| IBIS file stm32u575_585_lqfp144.ibs
[IBIS ver] 4.2
[File name] stm32u575_585_lqfp144.ibs
[File Rev] 1.0
[Date]   06-08-2021
[Source] Data Created at STMicroelectronics
[Notes]  File originated from ELDO simulations.
[Disclaimer]  This information is for modeling purpose only and is
   not guaranted. The information is subject to change without
   notice.
[Copyright] Copyright 2021 STMicroelectronics Inc.
|   Component stm32u575_585_lqfp144
[Component] stm32u575_585_lqfp144
[Manufacturer] STMicroelectronics
[Package]
| variable   typ   min   max
R_pkg   0   NA   NA
L_pkg   0   NA   NA
C_pkg   0   NA   NA
[Pin]   signal_name   model_name   R_pin   L_pin   C_pin   | Comment
1 PE2 io8_100m_hslv_ft 187.6E-3 9.4E-9 267.9E-15
2 PE3 io8_100m_hslv_tamp_ft 182.4E-3 9.1E-9 243.8E-15
3 PE4 io8_100m_hslv_tamp_ft 177.6E-3 8.7E-9 221.3E-15
4 PE5 io8_100m_hslv_tamp_ft 173.1E-3 8.4E-9 200.2E-15
5 PE6 io8_100m_hslv_tamp_ft 168.9E-3 8.1E-9 180.5E-15
6 VBAT POWER 165.0E-3 7.8E-9 162.3E-15
7 PC13 io8_100m_ft_v33 161.5E-3 7.6E-9 145.6E-15
8 PC14-OSC32_IN io8_100m_ft 158.2E-3 7.4E-9 130.3E-15
9 PC15-OSC32_OUT io8_100m_ft 155.2E-3 7.2E-9 116.4E-15
10 PF0 io8_100m_hslv_ft 152.6E-3 7.0E-9 104.1E-15
11 PF1 io8_100m_hslv_ft 150.3E-3 6.8E-9 93.2E-15
12 PF2 io8_100m_hslv_ft 148.2E-3 6.7E-9 83.7E-15
13 PF3 io8_100m_hslv_ft 146.5E-3 6.5E-9 75.7E-15
14 PF4 io8_166m_hslv_ft 145.1E-3 6.4E-9 69.1E-15
15 PF5 io8_166m_hslv_ft 144.1E-3 6.4E-9 64.0E-15
16 VSS GND 143.3E-3 6.3E-9 60.4E-15
17 VDD POWER 142.8E-3 6.3E-9 58.2E-15
18 PF6 io8_100m_hslv_ft 142.7E-3 6.3E-9 57.5E-15
19 PF7 io8_100m_hslv_ft 142.7E-3 6.3E-9 57.5E-15
20 PF8 io8_100m_hslv_ft 142.8E-3 6.3E-9 58.2E-15
21 PF9 io8_100m_hslv_ft 143.3E-3 6.3E-9 60.4E-15
22 PF10 io8_166m_hslv_ft 144.1E-3 6.4E-9 64.0E-15
23 PH0-OSC_IN io8_100m_ft 145.1E-3 6.4E-9 69.1E-15
24 PH1-OSC_OUT io8_100m_ft 146.5E-3 6.5E-9 75.7E-15
25 NRST nc 148.2E-3 6.7E-9 83.7E-15
26 PC0 io8_100m_hslv_ft 150.3E-3 6.8E-9 93.2E-15
27 PC1 io8_166m_hslv_i2c_ft 152.6E-3 7.0E-9 104.1E-15
28 PC2 io8_100m_hslv_ft 155.2E-3 7.2E-9 116.4E-15
29 PC3 io8_100m_hslv_ft 158.2E-3 7.4E-9 130.3E-15
30 VSSA GND 161.5E-3 7.6E-9 145.6E-15
31 VREF- GND 165.0E-3 7.8E-9 162.3E-15
32 VREF+ POWER 168.9E-3 8.1E-9 180.5E-15
33 VDDA POWER 173.1E-3 8.4E-9 200.2E-15
34 PA0 io8_100m_hslv_tamp_ft 177.6E-3 8.7E-9 221.3E-15
35 PA1 io8_100m_hslv_tamp_ft 182.4E-3 9.1E-9 243.8E-15
36 PA2 io8_100m_hslv_ft 187.6E-3 9.4E-9 267.9E-15
37 PA3 io8_166m_hslv_ft 187.6E-3 9.4E-9 267.9E-15
38 VSS GND 182.4E-3 9.1E-9 243.8E-15
39 VDD POWER 177.6E-3 8.7E-9 221.3E-15
40 PA4 io8_100m_hslv_ft 173.1E-3 8.4E-9 200.2E-15
41 PA5 io8_100m_ft 168.9E-3 8.1E-9 180.5E-15
42 PA6 io8_100m_hslv_ft 165.0E-3 7.8E-9 162.3E-15
43 PA7 io8_100m_hslv_ft 161.5E-3 7.6E-9 145.6E-15
44 PC4 io8_100m_hslv_ft 158.2E-3 7.4E-9 130.3E-15
45 PC5 io8_100m_tamp_ft 155.2E-3 7.2E-9 116.4E-15
46 PB0 io8_100m_hslv_ft 152.6E-3 7.0E-9 104.1E-15
47 PB1 io8_100m_hslv_ft 150.3E-3 6.8E-9 93.2E-15
48 PB2 io8_100m_hslv_tamp_ft 148.2E-3 6.7E-9 83.7E-15
49 PF11 io8_166m_hslv_ft 146.5E-3 6.5E-9 75.7E-15
50 PF12 io8_100m_hslv_ft 145.1E-3 6.4E-9 69.1E-15
51 VSS GND 144.1E-3 6.4E-9 64.0E-15
52 VDD POWER 143.3E-3 6.3E-9 60.4E-15
53 PF13 io8_100m_hslv_ft 142.8E-3 6.3E-9 58.2E-15
54 PF14 io8_100m_hslv_ft 142.7E-3 6.3E-9 57.5E-15
55 PF15 io8_100m_hslv_ft 142.7E-3 6.3E-9 57.5E-15
56 PG0 io8_100m_hslv_ft 142.8E-3 6.3E-9 58.2E-15
57 PG1 io8_100m_hslv_ft 143.3E-3 6.3E-9 60.4E-15
58 PE7 io8_100m_hslv_ft 144.1E-3 6.4E-9 64.0E-15
59 PE8 io8_100m_hslv_ft 145.1E-3 6.4E-9 69.1E-15
60 PE9 io8_166m_hslv_ft 146.5E-3 6.5E-9 75.7E-15
61 VSS GND 148.2E-3 6.7E-9 83.7E-15
62 VDD POWER 150.3E-3 6.8E-9 93.2E-15
63 PE10 io8_166m_hslv_ft 152.6E-3 7.0E-9 104.1E-15
64 PE11 io8_100m_hslv_ft 155.2E-3 7.2E-9 116.4E-15
65 PE12 io8_100m_hslv_ft 158.2E-3 7.4E-9 130.3E-15
66 PE13 io8_100m_hslv_ft 161.5E-3 7.6E-9 145.6E-15
67 PE14 io8_100m_hslv_ft 165.0E-3 7.8E-9 162.3E-15
68 PE15 io8_100m_hslv_ft 168.9E-3 8.1E-9 180.5E-15
69 PB10 io8_166m_hslv_i2c_ft 173.1E-3 8.4E-9 200.2E-15
70 VCAP POWER 177.6E-3 8.7E-9 221.3E-15
71 VSS GND 182.4E-3 9.1E-9 243.8E-15
72 VDD POWER 187.6E-3 9.4E-9 267.9E-15
73 PB12 io8_166m_hslv_ft 187.6E-3 9.4E-9 267.9E-15
74 PB13 io8_100m_i2c_ft 182.4E-3 9.1E-9 243.8E-15
75 PB14 io8_100m_i2c_ft 177.6E-3 8.7E-9 221.3E-15
76 PB15 nc 173.1E-3 8.4E-9 200.2E-15
77 PD8 io8_100m_hslv_ft 168.9E-3 8.1E-9 180.5E-15
78 PD9 io8_100m_hslv_ft 165.0E-3 7.8E-9 162.3E-15
79 PD10 io8_100m_hslv_ft 161.5E-3 7.6E-9 145.6E-15
80 PD11 io8_100m_hslv_ft 158.2E-3 7.4E-9 130.3E-15
81 PD12 io8_100m_hslv_ft 155.2E-3 7.2E-9 116.4E-15
82 PD13 io8_100m_hslv_ft 152.6E-3 7.0E-9 104.1E-15
83 VSS GND 150.3E-3 6.8E-9 93.2E-15
84 VDD POWER 148.2E-3 6.7E-9 83.7E-15
85 PD14 io8_100m_hslv_ft 146.5E-3 6.5E-9 75.7E-15
86 PD15 io8_100m_hslv_ft 145.1E-3 6.4E-9 69.1E-15
87 PG2 io8_100m_hslv_ft 144.1E-3 6.4E-9 64.0E-15
88 PG3 io8_100m_hslv_ft 143.3E-3 6.3E-9 60.4E-15
89 PG4 io8_100m_hslv_ft 142.8E-3 6.3E-9 58.2E-15
90 PG5 io8_100m_hslv_ft 142.7E-3 6.3E-9 57.5E-15
91 PG6 io8_100m_hslv_ft 142.7E-3 6.3E-9 57.5E-15
92 PG7 io8_100m_hslv_ft 142.8E-3 6.3E-9 58.2E-15
93 PG8 io8_100m_i2c_ft 143.3E-3 6.3E-9 60.4E-15
94 VSS GND 144.1E-3 6.4E-9 64.0E-15
95 VDDIO2 POWER 145.1E-3 6.4E-9 69.1E-15
96 PC6 io8_100m_ft 146.5E-3 6.5E-9 75.7E-15
97 PC7 io8_100m_ft 148.2E-3 6.7E-9 83.7E-15
98 PC8 io8_100m_ft 150.3E-3 6.8E-9 93.2E-15
99 PC9 io8_100m_ft 152.6E-3 7.0E-9 104.1E-15
100 PA8 io8_166m_hslv_ft 155.2E-3 7.2E-9 116.4E-15
101 PA9 io8_100m_usb_vbus_ft 158.2E-3 7.4E-9 130.3E-15
102 PA10 io8_100m_usb_id 161.5E-3 7.6E-9 145.6E-15
103 PA11 io8_usb_ft 165.0E-3 7.8E-9 162.3E-15
104 PA12 io8_usb_ft 168.9E-3 8.1E-9 180.5E-15
105 PA13 io8_100m_ft 173.1E-3 8.4E-9 200.2E-15
106 VDDUSB POWER 177.6E-3 8.7E-9 221.3E-15
107 VSS GND 182.4E-3 9.1E-9 243.8E-15
108 VDD POWER 187.6E-3 9.4E-9 267.9E-15
109 PA14 io8_100m_ft 187.6E-3 9.4E-9 267.9E-15
110 PA15 nc 182.4E-3 9.1E-9 243.8E-15
111 PC10 io8_100m_ft 177.6E-3 8.7E-9 221.3E-15
112 PC11 io8_100m_hslv_ft 173.1E-3 8.4E-9 200.2E-15
113 PC12 io8_166m_hslv_ft 168.9E-3 8.1E-9 180.5E-15
114 PD0 io8_100m_hslv_ft 165.0E-3 7.8E-9 162.3E-15
115 PD1 io8_100m_hslv_ft 161.5E-3 7.6E-9 145.6E-15
116 PD2 io8_100m_ft 158.2E-3 7.4E-9 130.3E-15
117 PD3 io8_166m_hslv_ft 155.2E-3 7.2E-9 116.4E-15
118 PD4 io8_100m_hslv_ft 152.6E-3 7.0E-9 104.1E-15
119 PD5 io8_100m_hslv_ft 150.3E-3 6.8E-9 93.2E-15
120 VSS GND 148.2E-3 6.7E-9 83.7E-15
121 VDD POWER 146.5E-3 6.5E-9 75.7E-15
122 PD6 io8_166m_hslv_ft 145.1E-3 6.4E-9 69.1E-15
123 PD7 io8_100m_hslv_ft 144.1E-3 6.4E-9 64.0E-15
124 PG9 io8_100m_hslv_ft 143.3E-3 6.3E-9 60.4E-15
125 PG10 io8_100m_hslv_ft 142.8E-3 6.3E-9 58.2E-15
126 PG11 io8_100m_hslv_ft 142.7E-3 6.3E-9 57.5E-15
127 PG12 io8_100m_hslv_ft 142.7E-3 6.3E-9 57.5E-15
128 PG13 io8_100m_hslv_ft 142.8E-3 6.3E-9 58.2E-15
129 PG14 io8_100m_hslv_ft 143.3E-3 6.3E-9 60.4E-15
130 VSS GND 144.1E-3 6.4E-9 64.0E-15
131 VDDIO2 POWER 145.1E-3 6.4E-9 69.1E-15
132 PG15 io8_100m_hslv_ft 146.5E-3 6.5E-9 75.7E-15
133 PB3 io8_100m_i2c_ft 148.2E-3 6.7E-9 83.7E-15
134 PB4 io8_100m_i2c_ft 150.3E-3 6.8E-9 93.2E-15
135 PB5 io8_166m_hslv_ft 152.6E-3 7.0E-9 104.1E-15
136 PB6 io8_100m_i2c_ft 155.2E-3 7.2E-9 116.4E-15
137 PB7 io8_166m_hslv_i2c_ft 158.2E-3 7.4E-9 130.3E-15
138 PH3-BOOT0 io8_100m_ft 161.5E-3 7.6E-9 145.6E-15
139 PB8 io8_100m_i2c_ft 165.0E-3 7.8E-9 162.3E-15
140 PB9 io8_100m_i2c_ft 168.9E-3 8.1E-9 180.5E-15
141 PE0 io8_100m_hslv_ft 173.1E-3 8.4E-9 200.2E-15
142 PE1 io8_100m_hslv_ft 177.6E-3 8.7E-9 221.3E-15
143 VSS GND 182.4E-3 9.1E-9 243.8E-15
144 VDD POWER 187.6E-3 9.4E-9 267.9E-15
[Model Selector] io8_100m_ft
io8_100m_ft_hs_1v2  "IO8_FT 100MHz high speed @ 1.2V"
io8_100m_ft_hs_pu_1v2  "IO8_FT 100MHz high speed @ 1.2V pullup"
io8_100m_ft_hs_pd_1v2  "IO8_FT 100MHz high speed @ 1.2V pulldown"
io8_100m_ft_fs_1v2  "IO8_FT 100MHz fast speed @ 1.2V"
io8_100m_ft_fs_pu_1v2  "IO8_FT 100MHz fast speed @ 1.2V pullup"
io8_100m_ft_fs_pd_1v2  "IO8_FT 100MHz fast speed @ 1.2V pulldown"
io8_100m_ft_ms_1v2  "IO8_FT 100MHz med speed @ 1.2V"
io8_100m_ft_ms_pu_1v2  "IO8_FT 100MHz med speed @ 1.2V pullup"
io8_100m_ft_ms_pd_1v2  "IO8_FT 100MHz med speed @ 1.2V pulldown"
io8_100m_ft_ls_1v2  "IO8_FT 100MHz low speed @ 1.2V"
io8_100m_ft_ls_pu_1v2  "IO8_FT 100MHz low speed @ 1.2V pullup"
io8_100m_ft_ls_pd_1v2  "IO8_FT 100MHz low speed @ 1.2V pulldown"
io8_100m_ft_hs_1v8  "IO8_FT 100MHz high speed @ 1.8V"
io8_100m_ft_hs_pu_1v8  "IO8_FT 100MHz high speed @ 1.8V pullup"
io8_100m_ft_hs_pd_1v8  "IO8_FT 100MHz high speed @ 1.8V pulldown"
io8_100m_ft_fs_1v8  "IO8_FT 100MHz fast speed @ 1.8V"
io8_100m_ft_fs_pu_1v8  "IO8_FT 100MHz fast speed @ 1.8V pullup"
io8_100m_ft_fs_pd_1v8  "IO8_FT 100MHz fast speed @ 1.8V pulldown"
io8_100m_ft_ms_1v8  "IO8_FT 100MHz med speed @ 1.8V"
io8_100m_ft_ms_pu_1v8  "IO8_FT 100MHz med speed @ 1.8V pullup"
io8_100m_ft_ms_pd_1v8  "IO8_FT 100MHz med speed @ 1.8V pulldown"
io8_100m_ft_ls_1v8  "IO8_FT 100MHz low speed @ 1.8V"
io8_100m_ft_ls_pu_1v8  "IO8_FT 100MHz low speed @ 1.8V pullup"
io8_100m_ft_ls_pd_1v8  "IO8_FT 100MHz low speed @ 1.8V pulldown"
io8_100m_ft_hs_3v3  "IO8_FT 100MHz high speed @ 3.3V"
io8_100m_ft_hs_pu_3v3  "IO8_FT 100MHz high speed @ 3.3V pullup"
io8_100m_ft_hs_pd_3v3  "IO8_FT 100MHz high speed @ 3.3V pulldown"
io8_100m_ft_fs_3v3  "IO8_FT 100MHz fast speed @ 3.3V"
io8_100m_ft_fs_pu_3v3  "IO8_FT 100MHz fast speed @ 3.3V pullup"
io8_100m_ft_fs_pd_3v3  "IO8_FT 100MHz fast speed @ 3.3V pulldown"
io8_100m_ft_ms_3v3  "IO8_FT 100MHz med speed @ 3.3V"
io8_100m_ft_ms_pu_3v3  "IO8_FT 100MHz med speed @ 3.3V pullup"
io8_100m_ft_ms_pd_3v3  "IO8_FT 100MHz med speed @ 3.3V pulldown"
io8_100m_ft_ls_3v3  "IO8_FT 100MHz low speed @ 3.3V"
io8_100m_ft_ls_pu_3v3  "IO8_FT 100MHz low speed @ 3.3V pullup"
io8_100m_ft_ls_pd_3v3  "IO8_FT 100MHz low speed @ 3.3V pulldown"
[Model Selector] io8_100m_hslv_ft
io8_100m_ft_hs_1v2  "IO8_FT 100MHz high speed @ 1.2V"
io8_100m_ft_hs_pu_1v2  "IO8_FT 100MHz high speed @ 1.2V pullup"
io8_100m_ft_hs_pd_1v2  "IO8_FT 100MHz high speed @ 1.2V pulldown"
io8_100m_ft_fs_1v2  "IO8_FT 100MHz fast speed @ 1.2V"
io8_100m_ft_fs_pu_1v2  "IO8_FT 100MHz fast speed @ 1.2V pullup"
io8_100m_ft_fs_pd_1v2  "IO8_FT 100MHz fast speed @ 1.2V pulldown"
io8_100m_ft_ms_1v2  "IO8_FT 100MHz med speed @ 1.2V"
io8_100m_ft_ms_pu_1v2  "IO8_FT 100MHz med speed @ 1.2V pullup"
io8_100m_ft_ms_pd_1v2  "IO8_FT 100MHz med speed @ 1.2V pulldown"
io8_100m_ft_ls_1v2  "IO8_FT 100MHz low speed @ 1.2V"
io8_100m_ft_ls_pu_1v2  "IO8_FT 100MHz low speed @ 1.2V pullup"
io8_100m_ft_ls_pd_1v2  "IO8_FT 100MHz low speed @ 1.2V pulldown"
io8_100m_ft_hs_1v8  "IO8_FT 100MHz high speed @ 1.8V"
io8_100m_ft_hs_pu_1v8  "IO8_FT 100MHz high speed @ 1.8V pullup"
io8_100m_ft_hs_pd_1v8  "IO8_FT 100MHz high speed @ 1.8V pulldown"
io8_100m_ft_fs_1v8  "IO8_FT 100MHz fast speed @ 1.8V"
io8_100m_ft_fs_pu_1v8  "IO8_FT 100MHz fast speed @ 1.8V pullup"
io8_100m_ft_fs_pd_1v8  "IO8_FT 100MHz fast speed @ 1.8V pulldown"
io8_100m_ft_ms_1v8  "IO8_FT 100MHz med speed @ 1.8V"
io8_100m_ft_ms_pu_1v8  "IO8_FT 100MHz med speed @ 1.8V pullup"
io8_100m_ft_ms_pd_1v8  "IO8_FT 100MHz med speed @ 1.8V pulldown"
io8_100m_ft_ls_1v8  "IO8_FT 100MHz low speed @ 1.8V"
io8_100m_ft_ls_pu_1v8  "IO8_FT 100MHz low speed @ 1.8V pullup"
io8_100m_ft_ls_pd_1v8  "IO8_FT 100MHz low speed @ 1.8V pulldown"
io8_100m_ft_hs_3v3  "IO8_FT 100MHz high speed @ 3.3V"
io8_100m_ft_hs_pu_3v3  "IO8_FT 100MHz high speed @ 3.3V pullup"
io8_100m_ft_hs_pd_3v3  "IO8_FT 100MHz high speed @ 3.3V pulldown"
io8_100m_ft_fs_3v3  "IO8_FT 100MHz fast speed @ 3.3V"
io8_100m_ft_fs_pu_3v3  "IO8_FT 100MHz fast speed @ 3.3V pullup"
io8_100m_ft_fs_pd_3v3  "IO8_FT 100MHz fast speed @ 3.3V pulldown"
io8_100m_ft_ms_3v3  "IO8_FT 100MHz med speed @ 3.3V"
io8_100m_ft_ms_pu_3v3  "IO8_FT 100MHz med speed @ 3.3V pullup"
io8_100m_ft_ms_pd_3v3  "IO8_FT 100MHz med speed @ 3.3V pulldown"
io8_100m_ft_ls_3v3  "IO8_FT 100MHz low speed @ 3.3V"
io8_100m_ft_ls_pu_3v3  "IO8_FT 100MHz low speed @ 3.3V pullup"
io8_100m_ft_ls_pd_3v3  "IO8_FT 100MHz low speed @ 3.3V pulldown"
io8_100m_hslv_ft_hs_1v2  "IO8_FT 100MHz HSLV high speed @ 1.2V"
io8_100m_hslv_ft_hs_pu_1v2  "IO8_FT 100MHz HSLV high speed @ 1.2V pullup"
io8_100m_hslv_ft_hs_pd_1v2  "IO8_FT 100MHz HSLV high speed @ 1.2V pulldown"
io8_100m_hslv_ft_fs_1v2  "IO8_FT 100MHz HSLV fast speed @ 1.2V"
io8_100m_hslv_ft_fs_pu_1v2  "IO8_FT 100MHz HSLV fast speed @ 1.2V pullup"
io8_100m_hslv_ft_fs_pd_1v2  "IO8_FT 100MHz HSLV fast speed @ 1.2V pulldown"
io8_100m_hslv_ft_ms_1v2  "IO8_FT 100MHz HSLV med speed @ 1.2V"
io8_100m_hslv_ft_ms_pu_1v2  "IO8_FT 100MHz HSLV med speed @ 1.2V pullup"
io8_100m_hslv_ft_ms_pd_1v2  "IO8_FT 100MHz HSLV med speed @ 1.2V pulldown"
io8_100m_hslv_ft_ls_1v2  "IO8_FT 100MHz HSLV low speed @ 1.2V"
io8_100m_hslv_ft_ls_pu_1v2  "IO8_FT 100MHz HSLV low speed @ 1.2V pullup"
io8_100m_hslv_ft_ls_pd_1v2  "IO8_FT 100MHz HSLV low speed @ 1.2V pulldown"
io8_100m_hslv_ft_hs_1v8  "IO8_FT 100MHz HSLV high speed @ 1.8V"
io8_100m_hslv_ft_hs_pu_1v8  "IO8_FT 100MHz HSLV high speed @ 1.8V pullup"
io8_100m_hslv_ft_hs_pd_1v8  "IO8_FT 100MHz HSLV high speed @ 1.8V pulldown"
io8_100m_hslv_ft_fs_1v8  "IO8_FT 100MHz HSLV fast speed @ 1.8V"
io8_100m_hslv_ft_fs_pu_1v8  "IO8_FT 100MHz HSLV fast speed @ 1.8V pullup"
io8_100m_hslv_ft_fs_pd_1v8  "IO8_FT 100MHz HSLV fast speed @ 1.8V pulldown"
io8_100m_hslv_ft_ms_1v8  "IO8_FT 100MHz HSLV med speed @ 1.8V"
io8_100m_hslv_ft_ms_pu_1v8  "IO8_FT 100MHz HSLV med speed @ 1.8V pullup"
io8_100m_hslv_ft_ms_pd_1v8  "IO8_FT 100MHz HSLV med speed @ 1.8V pulldown"
io8_100m_hslv_ft_ls_1v8  "IO8_FT 100MHz HSLV low speed @ 1.8V"
io8_100m_hslv_ft_ls_pu_1v8  "IO8_FT 100MHz HSLV low speed @ 1.8V pullup"
io8_100m_hslv_ft_ls_pd_1v8  "IO8_FT 100MHz HSLV low speed @ 1.8V pulldown"
io8_100m_hslv_ft_hs_2v5  "IO8_FT 100MHz HSLV high speed @ 2.5V"
io8_100m_hslv_ft_hs_pu_2v5  "IO8_FT 100MHz HSLV high speed @ 2.5V pullup"
io8_100m_hslv_ft_hs_pd_2v5  "IO8_FT 100MHz HSLV high speed @ 2.5V pulldown"
io8_100m_hslv_ft_fs_2v5  "IO8_FT 100MHz HSLV fast speed @ 2.5V"
io8_100m_hslv_ft_fs_pu_2v5  "IO8_FT 100MHz HSLV fast speed @ 2.5V pullup"
io8_100m_hslv_ft_fs_pd_2v5  "IO8_FT 100MHz HSLV fast speed @ 2.5V pulldown"
io8_100m_hslv_ft_ms_2v5  "IO8_FT 100MHz HSLV med speed @ 2.5V"
io8_100m_hslv_ft_ms_pu_2v5  "IO8_FT 100MHz HSLV med speed @ 2.5V pullup"
io8_100m_hslv_ft_ms_pd_2v5  "IO8_FT 100MHz HSLV med speed @ 2.5V pulldown"
io8_100m_hslv_ft_ls_2v5  "IO8_FT 100MHz HSLV low speed @ 2.5V"
io8_100m_hslv_ft_ls_pu_2v5  "IO8_FT 100MHz HSLV low speed @ 2.5V pullup"
io8_100m_hslv_ft_ls_pd_2v5  "IO8_FT 100MHz HSLV low speed @ 2.5V pulldown"
[Model Selector] io8_166m_hslv_ft
io8_166m_ft_hs_1v2  "IO8_FT 166MHz high speed @ 1.2V"
io8_166m_ft_hs_pu_1v2  "IO8_FT 166MHz high speed @ 1.2V pullup"
io8_166m_ft_hs_pd_1v2  "IO8_FT 166MHz high speed @ 1.2V pulldown"
io8_166m_ft_fs_1v2  "IO8_FT 166MHz fast speed @ 1.2V"
io8_166m_ft_fs_pu_1v2  "IO8_FT 166MHz fast speed @ 1.2V pullup"
io8_166m_ft_fs_pd_1v2  "IO8_FT 166MHz fast speed @ 1.2V pulldown"
io8_166m_ft_ms_1v2  "IO8_FT 166MHz med speed @ 1.2V"
io8_166m_ft_ms_pu_1v2  "IO8_FT 166MHz med speed @ 1.2V pullup"
io8_166m_ft_ms_pd_1v2  "IO8_FT 166MHz med speed @ 1.2V pulldown"
io8_166m_ft_ls_1v2  "IO8_FT 166MHz low speed @ 1.2V"
io8_166m_ft_ls_pu_1v2  "IO8_FT 166MHz low speed @ 1.2V pullup"
io8_166m_ft_ls_pd_1v2  "IO8_FT 166MHz low speed @ 1.2V pulldown"
io8_166m_ft_hs_1v8  "IO8_FT 166MHz high speed @ 1.8V"
io8_166m_ft_hs_pu_1v8  "IO8_FT 166MHz high speed @ 1.8V pullup"
io8_166m_ft_hs_pd_1v8  "IO8_FT 166MHz high speed @ 1.8V pulldown"
io8_166m_ft_fs_1v8  "IO8_FT 166MHz fast speed @ 1.8V"
io8_166m_ft_fs_pu_1v8  "IO8_FT 166MHz fast speed @ 1.8V pullup"
io8_166m_ft_fs_pd_1v8  "IO8_FT 166MHz fast speed @ 1.8V pulldown"
io8_166m_ft_ms_1v8  "IO8_FT 166MHz med speed @ 1.8V"
io8_166m_ft_ms_pu_1v8  "IO8_FT 166MHz med speed @ 1.8V pullup"
io8_166m_ft_ms_pd_1v8  "IO8_FT 166MHz med speed @ 1.8V pulldown"
io8_166m_ft_ls_1v8  "IO8_FT 166MHz low speed @ 1.8V"
io8_166m_ft_ls_pu_1v8  "IO8_FT 166MHz low speed @ 1.8V pullup"
io8_166m_ft_ls_pd_1v8  "IO8_FT 166MHz low speed @ 1.8V pulldown"
io8_166m_ft_hs_3v3  "IO8_FT 166MHz high speed @ 3.3V"
io8_166m_ft_hs_pu_3v3  "IO8_FT 166MHz high speed @ 3.3V pullup"
io8_166m_ft_hs_pd_3v3  "IO8_FT 166MHz high speed @ 3.3V pulldown"
io8_166m_ft_fs_3v3  "IO8_FT 166MHz fast speed @ 3.3V"
io8_166m_ft_fs_pu_3v3  "IO8_FT 166MHz fast speed @ 3.3V pullup"
io8_166m_ft_fs_pd_3v3  "IO8_FT 166MHz fast speed @ 3.3V pulldown"
io8_166m_ft_ms_3v3  "IO8_FT 166MHz med speed @ 3.3V"
io8_166m_ft_ms_pu_3v3  "IO8_FT 166MHz med speed @ 3.3V pullup"
io8_166m_ft_ms_pd_3v3  "IO8_FT 166MHz med speed @ 3.3V pulldown"
io8_166m_ft_ls_3v3  "IO8_FT 166MHz low speed @ 3.3V"
io8_166m_ft_ls_pu_3v3  "IO8_FT 166MHz low speed @ 3.3V pullup"
io8_166m_ft_ls_pd_3v3  "IO8_FT 166MHz low speed @ 3.3V pulldown"
io8_166m_hslv_ft_hs_1v2  "IO8_FT 166MHz HSLV high speed @ 1.2V"
io8_166m_hslv_ft_hs_pu_1v2  "IO8_FT 166MHz HSLV high speed @ 1.2V pullup"
io8_166m_hslv_ft_hs_pd_1v2  "IO8_FT 166MHz HSLV high speed @ 1.2V pulldown"
io8_166m_hslv_ft_fs_1v2  "IO8_FT 166MHz HSLV fast speed @ 1.2V"
io8_166m_hslv_ft_fs_pu_1v2  "IO8_FT 166MHz HSLV fast speed @ 1.2V pullup"
io8_166m_hslv_ft_fs_pd_1v2  "IO8_FT 166MHz HSLV fast speed @ 1.2V pulldown"
io8_166m_hslv_ft_ms_1v2  "IO8_FT 166MHz HSLV med speed @ 1.2V"
io8_166m_hslv_ft_ms_pu_1v2  "IO8_FT 166MHz HSLV med speed @ 1.2V pullup"
io8_166m_hslv_ft_ms_pd_1v2  "IO8_FT 166MHz HSLV med speed @ 1.2V pulldown"
io8_166m_hslv_ft_ls_1v2  "IO8_FT 166MHz HSLV low speed @ 1.2V"
io8_166m_hslv_ft_ls_pu_1v2  "IO8_FT 166MHz HSLV low speed @ 1.2V pullup"
io8_166m_hslv_ft_ls_pd_1v2  "IO8_FT 166MHz HSLV low speed @ 1.2V pulldown"
io8_166m_hslv_ft_hs_1v8  "IO8_FT 166MHz HSLV high speed @ 1.8V"
io8_166m_hslv_ft_hs_pu_1v8  "IO8_FT 166MHz HSLV high speed @ 1.8V pullup"
io8_166m_hslv_ft_hs_pd_1v8  "IO8_FT 166MHz HSLV high speed @ 1.8V pulldown"
io8_166m_hslv_ft_fs_1v8  "IO8_FT 166MHz HSLV fast speed @ 1.8V"
io8_166m_hslv_ft_fs_pu_1v8  "IO8_FT 166MHz HSLV fast speed @ 1.8V pullup"
io8_166m_hslv_ft_fs_pd_1v8  "IO8_FT 166MHz HSLV fast speed @ 1.8V pulldown"
io8_166m_hslv_ft_ms_1v8  "IO8_FT 166MHz HSLV med speed @ 1.8V"
io8_166m_hslv_ft_ms_pu_1v8  "IO8_FT 166MHz HSLV med speed @ 1.8V pullup"
io8_166m_hslv_ft_ms_pd_1v8  "IO8_FT 166MHz HSLV med speed @ 1.8V pulldown"
io8_166m_hslv_ft_ls_1v8  "IO8_FT 166MHz HSLV low speed @ 1.8V"
io8_166m_hslv_ft_ls_pu_1v8  "IO8_FT 166MHz HSLV low speed @ 1.8V pullup"
io8_166m_hslv_ft_ls_pd_1v8  "IO8_FT 166MHz HSLV low speed @ 1.8V pulldown"
io8_166m_hslv_ft_hs_2v5  "IO8_FT 166MHz HSLV high speed @ 2.5V"
io8_166m_hslv_ft_hs_pu_2v5  "IO8_FT 166MHz HSLV high speed @ 2.5V pullup"
io8_166m_hslv_ft_hs_pd_2v5  "IO8_FT 166MHz HSLV high speed @ 2.5V pulldown"
io8_166m_hslv_ft_fs_2v5  "IO8_FT 166MHz HSLV fast speed @ 2.5V"
io8_166m_hslv_ft_fs_pu_2v5  "IO8_FT 166MHz HSLV fast speed @ 2.5V pullup"
io8_166m_hslv_ft_fs_pd_2v5  "IO8_FT 166MHz HSLV fast speed @ 2.5V pulldown"
io8_166m_hslv_ft_ms_2v5  "IO8_FT 166MHz HSLV med speed @ 2.5V"
io8_166m_hslv_ft_ms_pu_2v5  "IO8_FT 166MHz HSLV med speed @ 2.5V pullup"
io8_166m_hslv_ft_ms_pd_2v5  "IO8_FT 166MHz HSLV med speed @ 2.5V pulldown"
io8_166m_hslv_ft_ls_2v5  "IO8_FT 166MHz HSLV low speed @ 2.5V"
io8_166m_hslv_ft_ls_pu_2v5  "IO8_FT 166MHz HSLV low speed @ 2.5V pullup"
io8_166m_hslv_ft_ls_pd_2v5  "IO8_FT 166MHz HSLV low speed @ 2.5V pulldown"
[Model Selector] io8_100m_ft_v33
io8_ft_v33_hs_1v2  "IO8_FT_V33 high speed @ 1.2V"
io8_ft_v33_hs_pu_1v2  "IO8_FT_V33 high speed @ 1.2V pullup"
io8_ft_v33_hs_pd_1v2  "IO8_FT_V33 high speed @ 1.2V pulldown"
io8_ft_v33_fs_1v2  "IO8_FT_V33 fast speed @ 1.2V"
io8_ft_v33_fs_pu_1v2  "IO8_FT_V33 fast speed @ 1.2V pullup"
io8_ft_v33_fs_pd_1v2  "IO8_FT_V33 fast speed @ 1.2V pulldown"
io8_ft_v33_ms_1v2  "IO8_FT_V33 med speed @ 1.2V"
io8_ft_v33_ms_pu_1v2  "IO8_FT_V33 med speed @ 1.2V pullup"
io8_ft_v33_ms_pd_1v2  "IO8_FT_V33 med speed @ 1.2V pulldown"
io8_ft_v33_ls_1v2  "IO8_FT_V33 low speed @ 1.2V"
io8_ft_v33_ls_pu_1v2  "IO8_FT_V33 low speed @ 1.2V pullup"
io8_ft_v33_ls_pd_1v2  "IO8_FT_V33 low speed @ 1.2V pulldown"
io8_ft_v33_hs_1v8  "IO8_FT_V33 high speed @ 1.8V"
io8_ft_v33_hs_pu_1v8  "IO8_FT_V33 high speed @ 1.8V pullup"
io8_ft_v33_hs_pd_1v8  "IO8_FT_V33 high speed @ 1.8V pulldown"
io8_ft_v33_fs_1v8  "IO8_FT_V33 fast speed @ 1.8V"
io8_ft_v33_fs_pu_1v8  "IO8_FT_V33 fast speed @ 1.8V pullup"
io8_ft_v33_fs_pd_1v8  "IO8_FT_V33 fast speed @ 1.8V pulldown"
io8_ft_v33_ms_1v8  "IO8_FT_V33 med speed @ 1.8V"
io8_ft_v33_ms_pu_1v8  "IO8_FT_V33 med speed @ 1.8V pullup"
io8_ft_v33_ms_pd_1v8  "IO8_FT_V33 med speed @ 1.8V pulldown"
io8_ft_v33_ls_1v8  "IO8_FT_V33 low speed @ 1.8V"
io8_ft_v33_ls_pu_1v8  "IO8_FT_V33 low speed @ 1.8V pullup"
io8_ft_v33_ls_pd_1v8  "IO8_FT_V33 low speed @ 1.8V pulldown"
io8_ft_v33_hs_3v3  "IO8_FT_V33 high speed @ 3.3V"
io8_ft_v33_hs_pu_3v3  "IO8_FT_V33 high speed @ 3.3V pullup"
io8_ft_v33_hs_pd_3v3  "IO8_FT_V33 high speed @ 3.3V pulldown"
io8_ft_v33_fs_3v3  "IO8_FT_V33 fast speed @ 3.3V"
io8_ft_v33_fs_pu_3v3  "IO8_FT_V33 fast speed @ 3.3V pullup"
io8_ft_v33_fs_pd_3v3  "IO8_FT_V33 fast speed @ 3.3V pulldown"
io8_ft_v33_ms_3v3  "IO8_FT_V33 med speed @ 3.3V"
io8_ft_v33_ms_pu_3v3  "IO8_FT_V33 med speed @ 3.3V pullup"
io8_ft_v33_ms_pd_3v3  "IO8_FT_V33 med speed @ 3.3V pulldown"
io8_ft_v33_ls_3v3  "IO8_FT_V33 low speed @ 3.3V"
io8_ft_v33_ls_pu_3v3  "IO8_FT_V33 low speed @ 3.3V pullup"
io8_ft_v33_ls_pd_3v3  "IO8_FT_V33 low speed @ 3.3V pulldown"
[Model Selector] io8_100m_tamp_ft
io8_100m_ft_hs_1v2  "IO8_FT 100MHz high speed @ 1.2V"
io8_100m_ft_hs_pu_1v2  "IO8_FT 100MHz high speed @ 1.2V pullup"
io8_100m_ft_hs_pd_1v2  "IO8_FT 100MHz high speed @ 1.2V pulldown"
io8_100m_ft_fs_1v2  "IO8_FT 100MHz fast speed @ 1.2V"
io8_100m_ft_fs_pu_1v2  "IO8_FT 100MHz fast speed @ 1.2V pullup"
io8_100m_ft_fs_pd_1v2  "IO8_FT 100MHz fast speed @ 1.2V pulldown"
io8_100m_ft_ms_1v2  "IO8_FT 100MHz med speed @ 1.2V"
io8_100m_ft_ms_pu_1v2  "IO8_FT 100MHz med speed @ 1.2V pullup"
io8_100m_ft_ms_pd_1v2  "IO8_FT 100MHz med speed @ 1.2V pulldown"
io8_100m_ft_ls_1v2  "IO8_FT 100MHz low speed @ 1.2V"
io8_100m_ft_ls_pu_1v2  "IO8_FT 100MHz low speed @ 1.2V pullup"
io8_100m_ft_ls_pd_1v2  "IO8_FT 100MHz low speed @ 1.2V pulldown"
io8_100m_ft_hs_1v8  "IO8_FT 100MHz high speed @ 1.8V"
io8_100m_ft_hs_pu_1v8  "IO8_FT 100MHz high speed @ 1.8V pullup"
io8_100m_ft_hs_pd_1v8  "IO8_FT 100MHz high speed @ 1.8V pulldown"
io8_100m_ft_fs_1v8  "IO8_FT 100MHz fast speed @ 1.8V"
io8_100m_ft_fs_pu_1v8  "IO8_FT 100MHz fast speed @ 1.8V pullup"
io8_100m_ft_fs_pd_1v8  "IO8_FT 100MHz fast speed @ 1.8V pulldown"
io8_100m_ft_ms_1v8  "IO8_FT 100MHz med speed @ 1.8V"
io8_100m_ft_ms_pu_1v8  "IO8_FT 100MHz med speed @ 1.8V pullup"
io8_100m_ft_ms_pd_1v8  "IO8_FT 100MHz med speed @ 1.8V pulldown"
io8_100m_ft_ls_1v8  "IO8_FT 100MHz low speed @ 1.8V"
io8_100m_ft_ls_pu_1v8  "IO8_FT 100MHz low speed @ 1.8V pullup"
io8_100m_ft_ls_pd_1v8  "IO8_FT 100MHz low speed @ 1.8V pulldown"
io8_100m_ft_hs_3v3  "IO8_FT 100MHz high speed @ 3.3V"
io8_100m_ft_hs_pu_3v3  "IO8_FT 100MHz high speed @ 3.3V pullup"
io8_100m_ft_hs_pd_3v3  "IO8_FT 100MHz high speed @ 3.3V pulldown"
io8_100m_ft_fs_3v3  "IO8_FT 100MHz fast speed @ 3.3V"
io8_100m_ft_fs_pu_3v3  "IO8_FT 100MHz fast speed @ 3.3V pullup"
io8_100m_ft_fs_pd_3v3  "IO8_FT 100MHz fast speed @ 3.3V pulldown"
io8_100m_ft_ms_3v3  "IO8_FT 100MHz med speed @ 3.3V"
io8_100m_ft_ms_pu_3v3  "IO8_FT 100MHz med speed @ 3.3V pullup"
io8_100m_ft_ms_pd_3v3  "IO8_FT 100MHz med speed @ 3.3V pulldown"
io8_100m_ft_ls_3v3  "IO8_FT 100MHz low speed @ 3.3V"
io8_100m_ft_ls_pu_3v3  "IO8_FT 100MHz low speed @ 3.3V pullup"
io8_100m_ft_ls_pd_3v3  "IO8_FT 100MHz low speed @ 3.3V pulldown"
io8_ft_v33_hs_1v2  "IO8_FT_V33 high speed @ 1.2V"
io8_ft_v33_hs_pu_1v2  "IO8_FT_V33 high speed @ 1.2V pullup"
io8_ft_v33_hs_pd_1v2  "IO8_FT_V33 high speed @ 1.2V pulldown"
io8_ft_v33_fs_1v2  "IO8_FT_V33 fast speed @ 1.2V"
io8_ft_v33_fs_pu_1v2  "IO8_FT_V33 fast speed @ 1.2V pullup"
io8_ft_v33_fs_pd_1v2  "IO8_FT_V33 fast speed @ 1.2V pulldown"
io8_ft_v33_ms_1v2  "IO8_FT_V33 med speed @ 1.2V"
io8_ft_v33_ms_pu_1v2  "IO8_FT_V33 med speed @ 1.2V pullup"
io8_ft_v33_ms_pd_1v2  "IO8_FT_V33 med speed @ 1.2V pulldown"
io8_ft_v33_ls_1v2  "IO8_FT_V33 low speed @ 1.2V"
io8_ft_v33_ls_pu_1v2  "IO8_FT_V33 low speed @ 1.2V pullup"
io8_ft_v33_ls_pd_1v2  "IO8_FT_V33 low speed @ 1.2V pulldown"
io8_ft_v33_hs_1v8  "IO8_FT_V33 high speed @ 1.8V"
io8_ft_v33_hs_pu_1v8  "IO8_FT_V33 high speed @ 1.8V pullup"
io8_ft_v33_hs_pd_1v8  "IO8_FT_V33 high speed @ 1.8V pulldown"
io8_ft_v33_fs_1v8  "IO8_FT_V33 fast speed @ 1.8V"
io8_ft_v33_fs_pu_1v8  "IO8_FT_V33 fast speed @ 1.8V pullup"
io8_ft_v33_fs_pd_1v8  "IO8_FT_V33 fast speed @ 1.8V pulldown"
io8_ft_v33_ms_1v8  "IO8_FT_V33 med speed @ 1.8V"
io8_ft_v33_ms_pu_1v8  "IO8_FT_V33 med speed @ 1.8V pullup"
io8_ft_v33_ms_pd_1v8  "IO8_FT_V33 med speed @ 1.8V pulldown"
io8_ft_v33_ls_1v8  "IO8_FT_V33 low speed @ 1.8V"
io8_ft_v33_ls_pu_1v8  "IO8_FT_V33 low speed @ 1.8V pullup"
io8_ft_v33_ls_pd_1v8  "IO8_FT_V33 low speed @ 1.8V pulldown"
io8_ft_v33_hs_3v3  "IO8_FT_V33 high speed @ 3.3V"
io8_ft_v33_hs_pu_3v3  "IO8_FT_V33 high speed @ 3.3V pullup"
io8_ft_v33_hs_pd_3v3  "IO8_FT_V33 high speed @ 3.3V pulldown"
io8_ft_v33_fs_3v3  "IO8_FT_V33 fast speed @ 3.3V"
io8_ft_v33_fs_pu_3v3  "IO8_FT_V33 fast speed @ 3.3V pullup"
io8_ft_v33_fs_pd_3v3  "IO8_FT_V33 fast speed @ 3.3V pulldown"
io8_ft_v33_ms_3v3  "IO8_FT_V33 med speed @ 3.3V"
io8_ft_v33_ms_pu_3v3  "IO8_FT_V33 med speed @ 3.3V pullup"
io8_ft_v33_ms_pd_3v3  "IO8_FT_V33 med speed @ 3.3V pulldown"
io8_ft_v33_ls_3v3  "IO8_FT_V33 low speed @ 3.3V"
io8_ft_v33_ls_pu_3v3  "IO8_FT_V33 low speed @ 3.3V pullup"
io8_ft_v33_ls_pd_3v3  "IO8_FT_V33 low speed @ 3.3V pulldown"
[Model Selector] io8_100m_hslv_tamp_ft
io8_100m_ft_hs_1v2  "IO8_FT 100MHz high speed @ 1.2V"
io8_100m_ft_hs_pu_1v2  "IO8_FT 100MHz high speed @ 1.2V pullup"
io8_100m_ft_hs_pd_1v2  "IO8_FT 100MHz high speed @ 1.2V pulldown"
io8_100m_ft_fs_1v2  "IO8_FT 100MHz fast speed @ 1.2V"
io8_100m_ft_fs_pu_1v2  "IO8_FT 100MHz fast speed @ 1.2V pullup"
io8_100m_ft_fs_pd_1v2  "IO8_FT 100MHz fast speed @ 1.2V pulldown"
io8_100m_ft_ms_1v2  "IO8_FT 100MHz med speed @ 1.2V"
io8_100m_ft_ms_pu_1v2  "IO8_FT 100MHz med speed @ 1.2V pullup"
io8_100m_ft_ms_pd_1v2  "IO8_FT 100MHz med speed @ 1.2V pulldown"
io8_100m_ft_ls_1v2  "IO8_FT 100MHz low speed @ 1.2V"
io8_100m_ft_ls_pu_1v2  "IO8_FT 100MHz low speed @ 1.2V pullup"
io8_100m_ft_ls_pd_1v2  "IO8_FT 100MHz low speed @ 1.2V pulldown"
io8_100m_ft_hs_1v8  "IO8_FT 100MHz high speed @ 1.8V"
io8_100m_ft_hs_pu_1v8  "IO8_FT 100MHz high speed @ 1.8V pullup"
io8_100m_ft_hs_pd_1v8  "IO8_FT 100MHz high speed @ 1.8V pulldown"
io8_100m_ft_fs_1v8  "IO8_FT 100MHz fast speed @ 1.8V"
io8_100m_ft_fs_pu_1v8  "IO8_FT 100MHz fast speed @ 1.8V pullup"
io8_100m_ft_fs_pd_1v8  "IO8_FT 100MHz fast speed @ 1.8V pulldown"
io8_100m_ft_ms_1v8  "IO8_FT 100MHz med speed @ 1.8V"
io8_100m_ft_ms_pu_1v8  "IO8_FT 100MHz med speed @ 1.8V pullup"
io8_100m_ft_ms_pd_1v8  "IO8_FT 100MHz med speed @ 1.8V pulldown"
io8_100m_ft_ls_1v8  "IO8_FT 100MHz low speed @ 1.8V"
io8_100m_ft_ls_pu_1v8  "IO8_FT 100MHz low speed @ 1.8V pullup"
io8_100m_ft_ls_pd_1v8  "IO8_FT 100MHz low speed @ 1.8V pulldown"
io8_100m_ft_hs_3v3  "IO8_FT 100MHz high speed @ 3.3V"
io8_100m_ft_hs_pu_3v3  "IO8_FT 100MHz high speed @ 3.3V pullup"
io8_100m_ft_hs_pd_3v3  "IO8_FT 100MHz high speed @ 3.3V pulldown"
io8_100m_ft_fs_3v3  "IO8_FT 100MHz fast speed @ 3.3V"
io8_100m_ft_fs_pu_3v3  "IO8_FT 100MHz fast speed @ 3.3V pullup"
io8_100m_ft_fs_pd_3v3  "IO8_FT 100MHz fast speed @ 3.3V pulldown"
io8_100m_ft_ms_3v3  "IO8_FT 100MHz med speed @ 3.3V"
io8_100m_ft_ms_pu_3v3  "IO8_FT 100MHz med speed @ 3.3V pullup"
io8_100m_ft_ms_pd_3v3  "IO8_FT 100MHz med speed @ 3.3V pulldown"
io8_100m_ft_ls_3v3  "IO8_FT 100MHz low speed @ 3.3V"
io8_100m_ft_ls_pu_3v3  "IO8_FT 100MHz low speed @ 3.3V pullup"
io8_100m_ft_ls_pd_3v3  "IO8_FT 100MHz low speed @ 3.3V pulldown"
io8_100m_hslv_ft_hs_1v2  "IO8_FT 100MHz HSLV high speed @ 1.2V"
io8_100m_hslv_ft_hs_pu_1v2  "IO8_FT 100MHz HSLV high speed @ 1.2V pullup"
io8_100m_hslv_ft_hs_pd_1v2  "IO8_FT 100MHz HSLV high speed @ 1.2V pulldown"
io8_100m_hslv_ft_fs_1v2  "IO8_FT 100MHz HSLV fast speed @ 1.2V"
io8_100m_hslv_ft_fs_pu_1v2  "IO8_FT 100MHz HSLV fast speed @ 1.2V pullup"
io8_100m_hslv_ft_fs_pd_1v2  "IO8_FT 100MHz HSLV fast speed @ 1.2V pulldown"
io8_100m_hslv_ft_ms_1v2  "IO8_FT 100MHz HSLV med speed @ 1.2V"
io8_100m_hslv_ft_ms_pu_1v2  "IO8_FT 100MHz HSLV med speed @ 1.2V pullup"
io8_100m_hslv_ft_ms_pd_1v2  "IO8_FT 100MHz HSLV med speed @ 1.2V pulldown"
io8_100m_hslv_ft_ls_1v2  "IO8_FT 100MHz HSLV low speed @ 1.2V"
io8_100m_hslv_ft_ls_pu_1v2  "IO8_FT 100MHz HSLV low speed @ 1.2V pullup"
io8_100m_hslv_ft_ls_pd_1v2  "IO8_FT 100MHz HSLV low speed @ 1.2V pulldown"
io8_100m_hslv_ft_hs_1v8  "IO8_FT 100MHz HSLV high speed @ 1.8V"
io8_100m_hslv_ft_hs_pu_1v8  "IO8_FT 100MHz HSLV high speed @ 1.8V pullup"
io8_100m_hslv_ft_hs_pd_1v8  "IO8_FT 100MHz HSLV high speed @ 1.8V pulldown"
io8_100m_hslv_ft_fs_1v8  "IO8_FT 100MHz HSLV fast speed @ 1.8V"
io8_100m_hslv_ft_fs_pu_1v8  "IO8_FT 100MHz HSLV fast speed @ 1.8V pullup"
io8_100m_hslv_ft_fs_pd_1v8  "IO8_FT 100MHz HSLV fast speed @ 1.8V pulldown"
io8_100m_hslv_ft_ms_1v8  "IO8_FT 100MHz HSLV med speed @ 1.8V"
io8_100m_hslv_ft_ms_pu_1v8  "IO8_FT 100MHz HSLV med speed @ 1.8V pullup"
io8_100m_hslv_ft_ms_pd_1v8  "IO8_FT 100MHz HSLV med speed @ 1.8V pulldown"
io8_100m_hslv_ft_ls_1v8  "IO8_FT 100MHz HSLV low speed @ 1.8V"
io8_100m_hslv_ft_ls_pu_1v8  "IO8_FT 100MHz HSLV low speed @ 1.8V pullup"
io8_100m_hslv_ft_ls_pd_1v8  "IO8_FT 100MHz HSLV low speed @ 1.8V pulldown"
io8_100m_hslv_ft_hs_2v5  "IO8_FT 100MHz HSLV high speed @ 2.5V"
io8_100m_hslv_ft_hs_pu_2v5  "IO8_FT 100MHz HSLV high speed @ 2.5V pullup"
io8_100m_hslv_ft_hs_pd_2v5  "IO8_FT 100MHz HSLV high speed @ 2.5V pulldown"
io8_100m_hslv_ft_fs_2v5  "IO8_FT 100MHz HSLV fast speed @ 2.5V"
io8_100m_hslv_ft_fs_pu_2v5  "IO8_FT 100MHz HSLV fast speed @ 2.5V pullup"
io8_100m_hslv_ft_fs_pd_2v5  "IO8_FT 100MHz HSLV fast speed @ 2.5V pulldown"
io8_100m_hslv_ft_ms_2v5  "IO8_FT 100MHz HSLV med speed @ 2.5V"
io8_100m_hslv_ft_ms_pu_2v5  "IO8_FT 100MHz HSLV med speed @ 2.5V pullup"
io8_100m_hslv_ft_ms_pd_2v5  "IO8_FT 100MHz HSLV med speed @ 2.5V pulldown"
io8_100m_hslv_ft_ls_2v5  "IO8_FT 100MHz HSLV low speed @ 2.5V"
io8_100m_hslv_ft_ls_pu_2v5  "IO8_FT 100MHz HSLV low speed @ 2.5V pullup"
io8_100m_hslv_ft_ls_pd_2v5  "IO8_FT 100MHz HSLV low speed @ 2.5V pulldown"
io8_ft_v33_hs_1v2  "IO8_FT_V33 high speed @ 1.2V"
io8_ft_v33_hs_pu_1v2  "IO8_FT_V33 high speed @ 1.2V pullup"
io8_ft_v33_hs_pd_1v2  "IO8_FT_V33 high speed @ 1.2V pulldown"
io8_ft_v33_fs_1v2  "IO8_FT_V33 fast speed @ 1.2V"
io8_ft_v33_fs_pu_1v2  "IO8_FT_V33 fast speed @ 1.2V pullup"
io8_ft_v33_fs_pd_1v2  "IO8_FT_V33 fast speed @ 1.2V pulldown"
io8_ft_v33_ms_1v2  "IO8_FT_V33 med speed @ 1.2V"
io8_ft_v33_ms_pu_1v2  "IO8_FT_V33 med speed @ 1.2V pullup"
io8_ft_v33_ms_pd_1v2  "IO8_FT_V33 med speed @ 1.2V pulldown"
io8_ft_v33_ls_1v2  "IO8_FT_V33 low speed @ 1.2V"
io8_ft_v33_ls_pu_1v2  "IO8_FT_V33 low speed @ 1.2V pullup"
io8_ft_v33_ls_pd_1v2  "IO8_FT_V33 low speed @ 1.2V pulldown"
io8_ft_v33_hs_1v8  "IO8_FT_V33 high speed @ 1.8V"
io8_ft_v33_hs_pu_1v8  "IO8_FT_V33 high speed @ 1.8V pullup"
io8_ft_v33_hs_pd_1v8  "IO8_FT_V33 high speed @ 1.8V pulldown"
io8_ft_v33_fs_1v8  "IO8_FT_V33 fast speed @ 1.8V"
io8_ft_v33_fs_pu_1v8  "IO8_FT_V33 fast speed @ 1.8V pullup"
io8_ft_v33_fs_pd_1v8  "IO8_FT_V33 fast speed @ 1.8V pulldown"
io8_ft_v33_ms_1v8  "IO8_FT_V33 med speed @ 1.8V"
io8_ft_v33_ms_pu_1v8  "IO8_FT_V33 med speed @ 1.8V pullup"
io8_ft_v33_ms_pd_1v8  "IO8_FT_V33 med speed @ 1.8V pulldown"
io8_ft_v33_ls_1v8  "IO8_FT_V33 low speed @ 1.8V"
io8_ft_v33_ls_pu_1v8  "IO8_FT_V33 low speed @ 1.8V pullup"
io8_ft_v33_ls_pd_1v8  "IO8_FT_V33 low speed @ 1.8V pulldown"
io8_ft_v33_hs_3v3  "IO8_FT_V33 high speed @ 3.3V"
io8_ft_v33_hs_pu_3v3  "IO8_FT_V33 high speed @ 3.3V pullup"
io8_ft_v33_hs_pd_3v3  "IO8_FT_V33 high speed @ 3.3V pulldown"
io8_ft_v33_fs_3v3  "IO8_FT_V33 fast speed @ 3.3V"
io8_ft_v33_fs_pu_3v3  "IO8_FT_V33 fast speed @ 3.3V pullup"
io8_ft_v33_fs_pd_3v3  "IO8_FT_V33 fast speed @ 3.3V pulldown"
io8_ft_v33_ms_3v3  "IO8_FT_V33 med speed @ 3.3V"
io8_ft_v33_ms_pu_3v3  "IO8_FT_V33 med speed @ 3.3V pullup"
io8_ft_v33_ms_pd_3v3  "IO8_FT_V33 med speed @ 3.3V pulldown"
io8_ft_v33_ls_3v3  "IO8_FT_V33 low speed @ 3.3V"
io8_ft_v33_ls_pu_3v3  "IO8_FT_V33 low speed @ 3.3V pullup"
io8_ft_v33_ls_pd_3v3  "IO8_FT_V33 low speed @ 3.3V pulldown"
[Model Selector] io8_100m_usb_id
io8_100m_ft_hs_1v2  "IO8_FT 100MHz high speed @ 1.2V"
io8_100m_ft_hs_pu_1v2  "IO8_FT 100MHz high speed @ 1.2V pullup"
io8_100m_ft_hs_pd_1v2  "IO8_FT 100MHz high speed @ 1.2V pulldown"
io8_100m_ft_fs_1v2  "IO8_FT 100MHz fast speed @ 1.2V"
io8_100m_ft_fs_pu_1v2  "IO8_FT 100MHz fast speed @ 1.2V pullup"
io8_100m_ft_fs_pd_1v2  "IO8_FT 100MHz fast speed @ 1.2V pulldown"
io8_100m_ft_ms_1v2  "IO8_FT 100MHz med speed @ 1.2V"
io8_100m_ft_ms_pu_1v2  "IO8_FT 100MHz med speed @ 1.2V pullup"
io8_100m_ft_ms_pd_1v2  "IO8_FT 100MHz med speed @ 1.2V pulldown"
io8_100m_ft_ls_1v2  "IO8_FT 100MHz low speed @ 1.2V"
io8_100m_ft_ls_pu_1v2  "IO8_FT 100MHz low speed @ 1.2V pullup"
io8_100m_ft_ls_pd_1v2  "IO8_FT 100MHz low speed @ 1.2V pulldown"
io8_100m_ft_hs_1v8  "IO8_FT 100MHz high speed @ 1.8V"
io8_100m_ft_hs_pu_1v8  "IO8_FT 100MHz high speed @ 1.8V pullup"
io8_100m_ft_hs_pd_1v8  "IO8_FT 100MHz high speed @ 1.8V pulldown"
io8_100m_ft_fs_1v8  "IO8_FT 100MHz fast speed @ 1.8V"
io8_100m_ft_fs_pu_1v8  "IO8_FT 100MHz fast speed @ 1.8V pullup"
io8_100m_ft_fs_pd_1v8  "IO8_FT 100MHz fast speed @ 1.8V pulldown"
io8_100m_ft_ms_1v8  "IO8_FT 100MHz med speed @ 1.8V"
io8_100m_ft_ms_pu_1v8  "IO8_FT 100MHz med speed @ 1.8V pullup"
io8_100m_ft_ms_pd_1v8  "IO8_FT 100MHz med speed @ 1.8V pulldown"
io8_100m_ft_ls_1v8  "IO8_FT 100MHz low speed @ 1.8V"
io8_100m_ft_ls_pu_1v8  "IO8_FT 100MHz low speed @ 1.8V pullup"
io8_100m_ft_ls_pd_1v8  "IO8_FT 100MHz low speed @ 1.8V pulldown"
io8_100m_ft_hs_3v3  "IO8_FT 100MHz high speed @ 3.3V"
io8_100m_ft_hs_pu_3v3  "IO8_FT 100MHz high speed @ 3.3V pullup"
io8_100m_ft_hs_pd_3v3  "IO8_FT 100MHz high speed @ 3.3V pulldown"
io8_100m_ft_fs_3v3  "IO8_FT 100MHz fast speed @ 3.3V"
io8_100m_ft_fs_pu_3v3  "IO8_FT 100MHz fast speed @ 3.3V pullup"
io8_100m_ft_fs_pd_3v3  "IO8_FT 100MHz fast speed @ 3.3V pulldown"
io8_100m_ft_ms_3v3  "IO8_FT 100MHz med speed @ 3.3V"
io8_100m_ft_ms_pu_3v3  "IO8_FT 100MHz med speed @ 3.3V pullup"
io8_100m_ft_ms_pd_3v3  "IO8_FT 100MHz med speed @ 3.3V pulldown"
io8_100m_ft_ls_3v3  "IO8_FT 100MHz low speed @ 3.3V"
io8_100m_ft_ls_pu_3v3  "IO8_FT 100MHz low speed @ 3.3V pullup"
io8_100m_ft_ls_pd_3v3  "IO8_FT 100MHz low speed @ 3.3V pulldown"
io8usb_id_nopu  "IOUSB ID @ 3.3V"
io8usb_id_pu  "IOUSB ID @ 3.3V pullup"
[Model Selector] io8_100m_usb_vbus_ft
io8_100m_ft_hs_1v2  "IO8_FT 100MHz high speed @ 1.2V"
io8_100m_ft_hs_pu_1v2  "IO8_FT 100MHz high speed @ 1.2V pullup"
io8_100m_ft_hs_pd_1v2  "IO8_FT 100MHz high speed @ 1.2V pulldown"
io8_100m_ft_fs_1v2  "IO8_FT 100MHz fast speed @ 1.2V"
io8_100m_ft_fs_pu_1v2  "IO8_FT 100MHz fast speed @ 1.2V pullup"
io8_100m_ft_fs_pd_1v2  "IO8_FT 100MHz fast speed @ 1.2V pulldown"
io8_100m_ft_ms_1v2  "IO8_FT 100MHz med speed @ 1.2V"
io8_100m_ft_ms_pu_1v2  "IO8_FT 100MHz med speed @ 1.2V pullup"
io8_100m_ft_ms_pd_1v2  "IO8_FT 100MHz med speed @ 1.2V pulldown"
io8_100m_ft_ls_1v2  "IO8_FT 100MHz low speed @ 1.2V"
io8_100m_ft_ls_pu_1v2  "IO8_FT 100MHz low speed @ 1.2V pullup"
io8_100m_ft_ls_pd_1v2  "IO8_FT 100MHz low speed @ 1.2V pulldown"
io8_100m_ft_hs_1v8  "IO8_FT 100MHz high speed @ 1.8V"
io8_100m_ft_hs_pu_1v8  "IO8_FT 100MHz high speed @ 1.8V pullup"
io8_100m_ft_hs_pd_1v8  "IO8_FT 100MHz high speed @ 1.8V pulldown"
io8_100m_ft_fs_1v8  "IO8_FT 100MHz fast speed @ 1.8V"
io8_100m_ft_fs_pu_1v8  "IO8_FT 100MHz fast speed @ 1.8V pullup"
io8_100m_ft_fs_pd_1v8  "IO8_FT 100MHz fast speed @ 1.8V pulldown"
io8_100m_ft_ms_1v8  "IO8_FT 100MHz med speed @ 1.8V"
io8_100m_ft_ms_pu_1v8  "IO8_FT 100MHz med speed @ 1.8V pullup"
io8_100m_ft_ms_pd_1v8  "IO8_FT 100MHz med speed @ 1.8V pulldown"
io8_100m_ft_ls_1v8  "IO8_FT 100MHz low speed @ 1.8V"
io8_100m_ft_ls_pu_1v8  "IO8_FT 100MHz low speed @ 1.8V pullup"
io8_100m_ft_ls_pd_1v8  "IO8_FT 100MHz low speed @ 1.8V pulldown"
io8_100m_ft_hs_3v3  "IO8_FT 100MHz high speed @ 3.3V"
io8_100m_ft_hs_pu_3v3  "IO8_FT 100MHz high speed @ 3.3V pullup"
io8_100m_ft_hs_pd_3v3  "IO8_FT 100MHz high speed @ 3.3V pulldown"
io8_100m_ft_fs_3v3  "IO8_FT 100MHz fast speed @ 3.3V"
io8_100m_ft_fs_pu_3v3  "IO8_FT 100MHz fast speed @ 3.3V pullup"
io8_100m_ft_fs_pd_3v3  "IO8_FT 100MHz fast speed @ 3.3V pulldown"
io8_100m_ft_ms_3v3  "IO8_FT 100MHz med speed @ 3.3V"
io8_100m_ft_ms_pu_3v3  "IO8_FT 100MHz med speed @ 3.3V pullup"
io8_100m_ft_ms_pd_3v3  "IO8_FT 100MHz med speed @ 3.3V pulldown"
io8_100m_ft_ls_3v3  "IO8_FT 100MHz low speed @ 3.3V"
io8_100m_ft_ls_pu_3v3  "IO8_FT 100MHz low speed @ 3.3V pullup"
io8_100m_ft_ls_pd_3v3  "IO8_FT 100MHz low speed @ 3.3V pulldown"
io8usb_adp "IOUSB ADP @ 3.3V"
io8usb_vbus "IOUSB VBUS @ 3.3V"
[Model Selector] io8_usb_ft
io8_100m_ft_hs_1v2  "IO8_FT 100MHz high speed @ 1.2V"
io8_100m_ft_hs_pu_1v2  "IO8_FT 100MHz high speed @ 1.2V pullup"
io8_100m_ft_hs_pd_1v2  "IO8_FT 100MHz high speed @ 1.2V pulldown"
io8_100m_ft_fs_1v2  "IO8_FT 100MHz fast speed @ 1.2V"
io8_100m_ft_fs_pu_1v2  "IO8_FT 100MHz fast speed @ 1.2V pullup"
io8_100m_ft_fs_pd_1v2  "IO8_FT 100MHz fast speed @ 1.2V pulldown"
io8_100m_ft_ms_1v2  "IO8_FT 100MHz med speed @ 1.2V"
io8_100m_ft_ms_pu_1v2  "IO8_FT 100MHz med speed @ 1.2V pullup"
io8_100m_ft_ms_pd_1v2  "IO8_FT 100MHz med speed @ 1.2V pulldown"
io8_100m_ft_ls_1v2  "IO8_FT 100MHz low speed @ 1.2V"
io8_100m_ft_ls_pu_1v2  "IO8_FT 100MHz low speed @ 1.2V pullup"
io8_100m_ft_ls_pd_1v2  "IO8_FT 100MHz low speed @ 1.2V pulldown"
io8_100m_ft_hs_1v8  "IO8_FT 100MHz high speed @ 1.8V"
io8_100m_ft_hs_pu_1v8  "IO8_FT 100MHz high speed @ 1.8V pullup"
io8_100m_ft_hs_pd_1v8  "IO8_FT 100MHz high speed @ 1.8V pulldown"
io8_100m_ft_fs_1v8  "IO8_FT 100MHz fast speed @ 1.8V"
io8_100m_ft_fs_pu_1v8  "IO8_FT 100MHz fast speed @ 1.8V pullup"
io8_100m_ft_fs_pd_1v8  "IO8_FT 100MHz fast speed @ 1.8V pulldown"
io8_100m_ft_ms_1v8  "IO8_FT 100MHz med speed @ 1.8V"
io8_100m_ft_ms_pu_1v8  "IO8_FT 100MHz med speed @ 1.8V pullup"
io8_100m_ft_ms_pd_1v8  "IO8_FT 100MHz med speed @ 1.8V pulldown"
io8_100m_ft_ls_1v8  "IO8_FT 100MHz low speed @ 1.8V"
io8_100m_ft_ls_pu_1v8  "IO8_FT 100MHz low speed @ 1.8V pullup"
io8_100m_ft_ls_pd_1v8  "IO8_FT 100MHz low speed @ 1.8V pulldown"
io8_100m_ft_hs_3v3  "IO8_FT 100MHz high speed @ 3.3V"
io8_100m_ft_hs_pu_3v3  "IO8_FT 100MHz high speed @ 3.3V pullup"
io8_100m_ft_hs_pd_3v3  "IO8_FT 100MHz high speed @ 3.3V pulldown"
io8_100m_ft_fs_3v3  "IO8_FT 100MHz fast speed @ 3.3V"
io8_100m_ft_fs_pu_3v3  "IO8_FT 100MHz fast speed @ 3.3V pullup"
io8_100m_ft_fs_pd_3v3  "IO8_FT 100MHz fast speed @ 3.3V pulldown"
io8_100m_ft_ms_3v3  "IO8_FT 100MHz med speed @ 3.3V"
io8_100m_ft_ms_pu_3v3  "IO8_FT 100MHz med speed @ 3.3V pullup"
io8_100m_ft_ms_pd_3v3  "IO8_FT 100MHz med speed @ 3.3V pulldown"
io8_100m_ft_ls_3v3  "IO8_FT 100MHz low speed @ 3.3V"
io8_100m_ft_ls_pu_3v3  "IO8_FT 100MHz low speed @ 3.3V pullup"
io8_100m_ft_ls_pd_3v3  "IO8_FT 100MHz low speed @ 3.3V pulldown"
io8_usb_fs_3v3  "IOUSB fast speed @ 3.3V"
io8_usb_fs_pu1_3v3  "IO8USB fast speed @ 3.3V pullup1"
io8_usb_fs_pd1_3v3  "IOUSB fast speed @ 3.3V pulldown1"
io8_usb_ls_3v3  "IOUSB low speed @ 3.3V"
io8_usb_ls_pu1_3v3  "IOUSB low speed @ 3.3V pullup1"
io8_usb_ls_pd1_3v3  "IOUSB low speed @ 3.3V pulldown1"
io8_usb_fs_pu2_3v3  "IOUSB fast speed @ 3.3V pullup2"
io8_usb_fs_pd2_3v3  "IOUSB fast speed @ 3.3V pulldown2"
io8_usb_ls_pu2_3v3  "IOUSB low speed @ 3.3V pullup2"
io8_usb_ls_pd2_3v3  "IOUSB low speed @ 3.3V pulldown2"
[Model Selector] io8_100m_i2c_ft
io8_100m_ft_hs_1v2  "IO8_FT 100MHz high speed @ 1.2V"
io8_100m_ft_hs_pu_1v2  "IO8_FT 100MHz high speed @ 1.2V pullup"
io8_100m_ft_hs_pd_1v2  "IO8_FT 100MHz high speed @ 1.2V pulldown"
io8_100m_ft_fs_1v2  "IO8_FT 100MHz fast speed @ 1.2V"
io8_100m_ft_fs_pu_1v2  "IO8_FT 100MHz fast speed @ 1.2V pullup"
io8_100m_ft_fs_pd_1v2  "IO8_FT 100MHz fast speed @ 1.2V pulldown"
io8_100m_ft_ms_1v2  "IO8_FT 100MHz med speed @ 1.2V"
io8_100m_ft_ms_pu_1v2  "IO8_FT 100MHz med speed @ 1.2V pullup"
io8_100m_ft_ms_pd_1v2  "IO8_FT 100MHz med speed @ 1.2V pulldown"
io8_100m_ft_ls_1v2  "IO8_FT 100MHz low speed @ 1.2V"
io8_100m_ft_ls_pu_1v2  "IO8_FT 100MHz low speed @ 1.2V pullup"
io8_100m_ft_ls_pd_1v2  "IO8_FT 100MHz low speed @ 1.2V pulldown"
io8_100m_ft_hs_1v8  "IO8_FT 100MHz high speed @ 1.8V"
io8_100m_ft_hs_pu_1v8  "IO8_FT 100MHz high speed @ 1.8V pullup"
io8_100m_ft_hs_pd_1v8  "IO8_FT 100MHz high speed @ 1.8V pulldown"
io8_100m_ft_fs_1v8  "IO8_FT 100MHz fast speed @ 1.8V"
io8_100m_ft_fs_pu_1v8  "IO8_FT 100MHz fast speed @ 1.8V pullup"
io8_100m_ft_fs_pd_1v8  "IO8_FT 100MHz fast speed @ 1.8V pulldown"
io8_100m_ft_ms_1v8  "IO8_FT 100MHz med speed @ 1.8V"
io8_100m_ft_ms_pu_1v8  "IO8_FT 100MHz med speed @ 1.8V pullup"
io8_100m_ft_ms_pd_1v8  "IO8_FT 100MHz med speed @ 1.8V pulldown"
io8_100m_ft_ls_1v8  "IO8_FT 100MHz low speed @ 1.8V"
io8_100m_ft_ls_pu_1v8  "IO8_FT 100MHz low speed @ 1.8V pullup"
io8_100m_ft_ls_pd_1v8  "IO8_FT 100MHz low speed @ 1.8V pulldown"
io8_100m_ft_hs_3v3  "IO8_FT 100MHz high speed @ 3.3V"
io8_100m_ft_hs_pu_3v3  "IO8_FT 100MHz high speed @ 3.3V pullup"
io8_100m_ft_hs_pd_3v3  "IO8_FT 100MHz high speed @ 3.3V pulldown"
io8_100m_ft_fs_3v3  "IO8_FT 100MHz fast speed @ 3.3V"
io8_100m_ft_fs_pu_3v3  "IO8_FT 100MHz fast speed @ 3.3V pullup"
io8_100m_ft_fs_pd_3v3  "IO8_FT 100MHz fast speed @ 3.3V pulldown"
io8_100m_ft_ms_3v3  "IO8_FT 100MHz med speed @ 3.3V"
io8_100m_ft_ms_pu_3v3  "IO8_FT 100MHz med speed @ 3.3V pullup"
io8_100m_ft_ms_pd_3v3  "IO8_FT 100MHz med speed @ 3.3V pulldown"
io8_100m_ft_ls_3v3  "IO8_FT 100MHz low speed @ 3.3V"
io8_100m_ft_ls_pu_3v3  "IO8_FT 100MHz low speed @ 3.3V pullup"
io8_100m_ft_ls_pd_3v3  "IO8_FT 100MHz low speed @ 3.3V pulldown"
io8_100m_i2c_ft_1v2  "IO8_FT 100MHz I2C @ 1.2V"
io8_100m_i2c_ft_pu_1v2  "IO8_FT 100MHz I2C @ 1.2V pullup"
io8_100m_i2c_ft_pd_1v2  "IO8_FT 100MHz I2C @ 1.2V pulldown"
io8_100m_i2c_ft_1v8  "IO8_FT 100MHz I2C @ 1.8V"
io8_100m_i2c_ft_pu_1v8  "IO8_FT 100MHz I2C @ 1.8V pullup"
io8_100m_i2c_ft_pd_1v8  "IO8_FT 100MHz I2C @ 1,8V pulldown"
io8_100m_i2c_ft_3v3  "IO8_FT 100MHz I2C @ 3.3V"
io8_100m_i2c_ft_pu_3v3  "IO8_FT 100MHz I2C HSLV @ 3.3V pullup"
io8_100m_i2c_ft_pd_3v3  "IO8_FT 100MHz I2C @ 3.3V pulldown"
[Model Selector] io8_166m_hslv_i2c_ft
io8_166m_ft_hs_1v2  "IO8_FT 166MHz high speed @ 1.2V"
io8_166m_ft_hs_pu_1v2  "IO8_FT 166MHz high speed @ 1.2V pullup"
io8_166m_ft_hs_pd_1v2  "IO8_FT 166MHz high speed @ 1.2V pulldown"
io8_166m_ft_fs_1v2  "IO8_FT 166MHz fast speed @ 1.2V"
io8_166m_ft_fs_pu_1v2  "IO8_FT 166MHz fast speed @ 1.2V pullup"
io8_166m_ft_fs_pd_1v2  "IO8_FT 166MHz fast speed @ 1.2V pulldown"
io8_166m_ft_ms_1v2  "IO8_FT 166MHz med speed @ 1.2V"
io8_166m_ft_ms_pu_1v2  "IO8_FT 166MHz med speed @ 1.2V pullup"
io8_166m_ft_ms_pd_1v2  "IO8_FT 166MHz med speed @ 1.2V pulldown"
io8_166m_ft_ls_1v2  "IO8_FT 166MHz low speed @ 1.2V"
io8_166m_ft_ls_pu_1v2  "IO8_FT 166MHz low speed @ 1.2V pullup"
io8_166m_ft_ls_pd_1v2  "IO8_FT 166MHz low speed @ 1.2V pulldown"
io8_166m_ft_hs_1v8  "IO8_FT 166MHz high speed @ 1.8V"
io8_166m_ft_hs_pu_1v8  "IO8_FT 166MHz high speed @ 1.8V pullup"
io8_166m_ft_hs_pd_1v8  "IO8_FT 166MHz high speed @ 1.8V pulldown"
io8_166m_ft_fs_1v8  "IO8_FT 166MHz fast speed @ 1.8V"
io8_166m_ft_fs_pu_1v8  "IO8_FT 166MHz fast speed @ 1.8V pullup"
io8_166m_ft_fs_pd_1v8  "IO8_FT 166MHz fast speed @ 1.8V pulldown"
io8_166m_ft_ms_1v8  "IO8_FT 166MHz med speed @ 1.8V"
io8_166m_ft_ms_pu_1v8  "IO8_FT 166MHz med speed @ 1.8V pullup"
io8_166m_ft_ms_pd_1v8  "IO8_FT 166MHz med speed @ 1.8V pulldown"
io8_166m_ft_ls_1v8  "IO8_FT 166MHz low speed @ 1.8V"
io8_166m_ft_ls_pu_1v8  "IO8_FT 166MHz low speed @ 1.8V pullup"
io8_166m_ft_ls_pd_1v8  "IO8_FT 166MHz low speed @ 1.8V pulldown"
io8_166m_ft_hs_3v3  "IO8_FT 166MHz high speed @ 3.3V"
io8_166m_ft_hs_pu_3v3  "IO8_FT 166MHz high speed @ 3.3V pullup"
io8_166m_ft_hs_pd_3v3  "IO8_FT 166MHz high speed @ 3.3V pulldown"
io8_166m_ft_fs_3v3  "IO8_FT 166MHz fast speed @ 3.3V"
io8_166m_ft_fs_pu_3v3  "IO8_FT 166MHz fast speed @ 3.3V pullup"
io8_166m_ft_fs_pd_3v3  "IO8_FT 166MHz fast speed @ 3.3V pulldown"
io8_166m_ft_ms_3v3  "IO8_FT 166MHz med speed @ 3.3V"
io8_166m_ft_ms_pu_3v3  "IO8_FT 166MHz med speed @ 3.3V pullup"
io8_166m_ft_ms_pd_3v3  "IO8_FT 166MHz med speed @ 3.3V pulldown"
io8_166m_ft_ls_3v3  "IO8_FT 166MHz low speed @ 3.3V"
io8_166m_ft_ls_pu_3v3  "IO8_FT 166MHz low speed @ 3.3V pullup"
io8_166m_ft_ls_pd_3v3  "IO8_FT 166MHz low speed @ 3.3V pulldown"
io8_166m_hslv_ft_hs_1v2  "IO8_FT 166MHz HSLV high speed @ 1.2V"
io8_166m_hslv_ft_hs_pu_1v2  "IO8_FT 166MHz HSLV high speed @ 1.2V pullup"
io8_166m_hslv_ft_hs_pd_1v2  "IO8_FT 166MHz HSLV high speed @ 1.2V pulldown"
io8_166m_hslv_ft_fs_1v2  "IO8_FT 166MHz HSLV fast speed @ 1.2V"
io8_166m_hslv_ft_fs_pu_1v2  "IO8_FT 166MHz HSLV fast speed @ 1.2V pullup"
io8_166m_hslv_ft_fs_pd_1v2  "IO8_FT 166MHz HSLV fast speed @ 1.2V pulldown"
io8_166m_hslv_ft_ms_1v2  "IO8_FT 166MHz HSLV med speed @ 1.2V"
io8_166m_hslv_ft_ms_pu_1v2  "IO8_FT 166MHz HSLV med speed @ 1.2V pullup"
io8_166m_hslv_ft_ms_pd_1v2  "IO8_FT 166MHz HSLV med speed @ 1.2V pulldown"
io8_166m_hslv_ft_ls_1v2  "IO8_FT 166MHz HSLV low speed @ 1.2V"
io8_166m_hslv_ft_ls_pu_1v2  "IO8_FT 166MHz HSLV low speed @ 1.2V pullup"
io8_166m_hslv_ft_ls_pd_1v2  "IO8_FT 166MHz HSLV low speed @ 1.2V pulldown"
io8_166m_hslv_ft_hs_1v8  "IO8_FT 166MHz HSLV high speed @ 1.8V"
io8_166m_hslv_ft_hs_pu_1v8  "IO8_FT 166MHz HSLV high speed @ 1.8V pullup"
io8_166m_hslv_ft_hs_pd_1v8  "IO8_FT 166MHz HSLV high speed @ 1.8V pulldown"
io8_166m_hslv_ft_fs_1v8  "IO8_FT 166MHz HSLV fast speed @ 1.8V"
io8_166m_hslv_ft_fs_pu_1v8  "IO8_FT 166MHz HSLV fast speed @ 1.8V pullup"
io8_166m_hslv_ft_fs_pd_1v8  "IO8_FT 166MHz HSLV fast speed @ 1.8V pulldown"
io8_166m_hslv_ft_ms_1v8  "IO8_FT 166MHz HSLV med speed @ 1.8V"
io8_166m_hslv_ft_ms_pu_1v8  "IO8_FT 166MHz HSLV med speed @ 1.8V pullup"
io8_166m_hslv_ft_ms_pd_1v8  "IO8_FT 166MHz HSLV med speed @ 1.8V pulldown"
io8_166m_hslv_ft_ls_1v8  "IO8_FT 166MHz HSLV low speed @ 1.8V"
io8_166m_hslv_ft_ls_pu_1v8  "IO8_FT 166MHz HSLV low speed @ 1.8V pullup"
io8_166m_hslv_ft_ls_pd_1v8  "IO8_FT 166MHz HSLV low speed @ 1.8V pulldown"
io8_166m_hslv_ft_hs_2v5  "IO8_FT 166MHz HSLV high speed @ 2.5V"
io8_166m_hslv_ft_hs_pu_2v5  "IO8_FT 166MHz HSLV high speed @ 2.5V pullup"
io8_166m_hslv_ft_hs_pd_2v5  "IO8_FT 166MHz HSLV high speed @ 2.5V pulldown"
io8_166m_hslv_ft_fs_2v5  "IO8_FT 166MHz HSLV fast speed @ 2.5V"
io8_166m_hslv_ft_fs_pu_2v5  "IO8_FT 166MHz HSLV fast speed @ 2.5V pullup"
io8_166m_hslv_ft_fs_pd_2v5  "IO8_FT 166MHz HSLV fast speed @ 2.5V pulldown"
io8_166m_hslv_ft_ms_2v5  "IO8_FT 166MHz HSLV med speed @ 2.5V"
io8_166m_hslv_ft_ms_pu_2v5  "IO8_FT 166MHz HSLV med speed @ 2.5V pullup"
io8_166m_hslv_ft_ms_pd_2v5  "IO8_FT 166MHz HSLV med speed @ 2.5V pulldown"
io8_166m_hslv_ft_ls_2v5  "IO8_FT 166MHz HSLV low speed @ 2.5V"
io8_166m_hslv_ft_ls_pu_2v5  "IO8_FT 166MHz HSLV low speed @ 2.5V pullup"
io8_166m_hslv_ft_ls_pd_2v5  "IO8_FT 166MHz HSLV low speed @ 2.5V pulldown"
io8_166m_i2c_ft_1v2  "IO8_FT 166MHz I2C @ 1.2V"
io8_166m_i2c_ft_pu_1v2  "IO8_FT 166MHz I2C @ 1.2V pullup"
io8_166m_i2c_ft_pd_1v2  "IO8_FT 166MHz I2C @ 1.2V pulldown"
io8_166m_i2c_ft_1v8  "IO8_FT 166MHz I2C @ 1.8V"
io8_166m_i2c_ft_pu_1v8  "IO8_FT 166MHz I2C @ 1.8V pullup"
io8_166m_i2c_ft_pd_1v8  "IO8_FT 166MHz I2C @ 1,8V pulldown"
io8_166m_i2c_ft_3v3  "IO8_FT 166MHz I2C @ 3.3V"
io8_166m_i2c_ft_pu_3v3  "IO8_FT 166MHz I2C HSLV @ 3.3V pullup"
io8_166m_i2c_ft_pd_3v3  "IO8_FT 166MHz I2C @ 3.3V pulldown"
| Models and submodels in the file (212): io8_100m_ft_hs_1v2 (I/O), io8_100m_ft_hs_pu_1v2 (I/O), io8_100m_ft_hs_pd_1v2 (I/O), io8_100m_ft_fs_1v2 (I/O), io8_100m_ft_fs_pu_1v2 (I/O), io8_100m_ft_fs_pd_1v2 (I/O), io8_100m_ft_ms_1v2 (I/O), io8_100m_ft_ms_pu_1v2 (I/O), io8_100m_ft_ms_pd_1v2 (I/O), io8_100m_ft_ls_1v2 (I/O), io8_100m_ft_ls_pu_1v2 (I/O), io8_100m_ft_ls_pd_1v2 (I/O), io8_100m_ft_hs_1v8 (I/O), io8_100m_ft_hs_pu_1v8 (I/O), io8_100m_ft_hs_pd_1v8 (I/O), io8_100m_ft_fs_1v8 (I/O), io8_100m_ft_fs_pu_1v8 (I/O), io8_100m_ft_fs_pd_1v8 (I/O), io8_100m_ft_ms_1v8 (I/O), io8_100m_ft_ms_pu_1v8 (I/O), io8_100m_ft_ms_pd_1v8 (I/O), io8_100m_ft_ls_1v8 (I/O), io8_100m_ft_ls_pu_1v8 (I/O), io8_100m_ft_ls_pd_1v8 (I/O), io8_100m_ft_hs_3v3 (I/O), io8_100m_ft_hs_pu_3v3 (I/O), io8_100m_ft_hs_pd_3v3 (I/O), io8_100m_ft_fs_3v3 (I/O), io8_100m_ft_fs_pu_3v3 (I/O), io8_100m_ft_fs_pd_3v3 (I/O), io8_100m_ft_ms_3v3 (I/O), io8_100m_ft_ms_pu_3v3 (I/O), io8_100m_ft_ms_pd_3v3 (I/O), io8_100m_ft_ls_3v3 (I/O), io8_100m_ft_ls_pu_3v3 (I/O), io8_100m_ft_ls_pd_3v3 (I/O), io8_100m_hslv_ft_hs_1v2 (I/O), io8_100m_hslv_ft_hs_pu_1v2 (I/O), io8_100m_hslv_ft_hs_pd_1v2 (I/O), io8_100m_hslv_ft_fs_1v2 (I/O), io8_100m_hslv_ft_fs_pu_1v2 (I/O), io8_100m_hslv_ft_fs_pd_1v2 (I/O), io8_100m_hslv_ft_ms_1v2 (I/O), io8_100m_hslv_ft_ms_pu_1v2 (I/O), io8_100m_hslv_ft_ms_pd_1v2 (I/O), io8_100m_hslv_ft_ls_1v2 (I/O), io8_100m_hslv_ft_ls_pu_1v2 (I/O), io8_100m_hslv_ft_ls_pd_1v2 (I/O), io8_100m_hslv_ft_hs_1v8 (I/O), io8_100m_hslv_ft_hs_pu_1v8 (I/O), io8_100m_hslv_ft_hs_pd_1v8 (I/O), io8_100m_hslv_ft_fs_1v8 (I/O), io8_100m_hslv_ft_fs_pu_1v8 (I/O), io8_100m_hslv_ft_fs_pd_1v8 (I/O), io8_100m_hslv_ft_ms_1v8 (I/O), io8_100m_hslv_ft_ms_pu_1v8 (I/O), io8_100m_hslv_ft_ms_pd_1v8 (I/O), io8_100m_hslv_ft_ls_1v8 (I/O), io8_100m_hslv_ft_ls_pu_1v8 (I/O), io8_100m_hslv_ft_ls_pd_1v8 (I/O), io8_100m_hslv_ft_hs_2v5 (I/O), io8_100m_hslv_ft_hs_pu_2v5 (I/O), io8_100m_hslv_ft_hs_pd_2v5 (I/O), io8_100m_hslv_ft_fs_2v5 (I/O), io8_100m_hslv_ft_fs_pu_2v5 (I/O), io8_100m_hslv_ft_fs_pd_2v5 (I/O), io8_100m_hslv_ft_ms_2v5 (I/O), io8_100m_hslv_ft_ms_pu_2v5 (I/O), io8_100m_hslv_ft_ms_pd_2v5 (I/O), io8_100m_hslv_ft_ls_2v5 (I/O), io8_100m_hslv_ft_ls_pu_2v5 (I/O), io8_100m_hslv_ft_ls_pd_2v5 (I/O), io8_166m_ft_hs_1v2 (I/O), io8_166m_ft_hs_pu_1v2 (I/O), io8_166m_ft_hs_pd_1v2 (I/O), io8_166m_ft_fs_1v2 (I/O), io8_166m_ft_fs_pu_1v2 (I/O), io8_166m_ft_fs_pd_1v2 (I/O), io8_166m_ft_ms_1v2 (I/O), io8_166m_ft_ms_pu_1v2 (I/O)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
